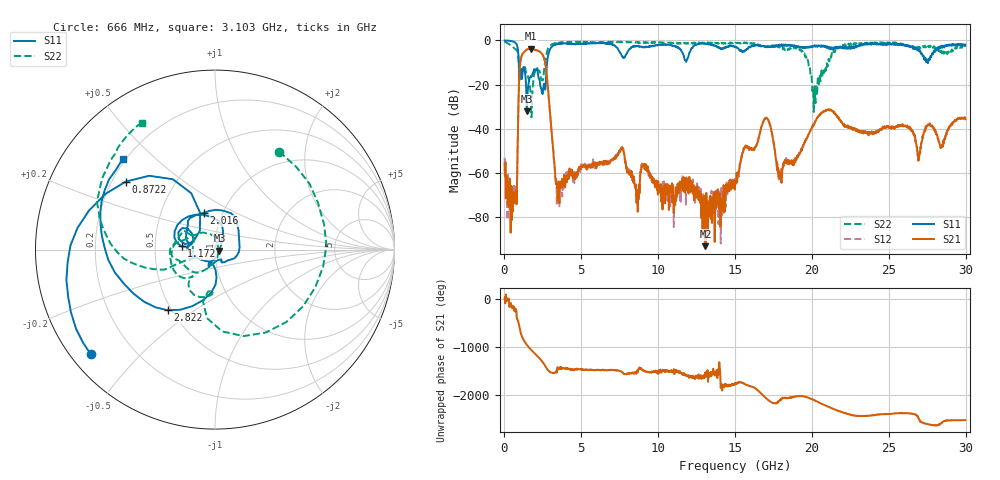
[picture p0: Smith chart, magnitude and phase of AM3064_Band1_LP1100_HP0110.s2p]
# Hz S DB R 50.0
!freq dBS11 angS11 dBS21 angS21 dBS12 angS12 dBS22 angS22
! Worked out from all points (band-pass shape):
!   1600 points, 10 MHz to 29.98 GHz, reference 50 ohm
!   highest |S21| = -3.79 dB at 1.697 GHz (marker M1); lowest = -93.0 dB at 13.07 GHz (marker M2)
!   |S21| within 3 dB of the highest: 1.133 GHz to 2.5 GHz (1.367 GHz wide, 75.3 % of centre)
!   lowest |S11| = -32.0 dB at 1.453 GHz (marker M3), VSWR 1.05, Z = 52.5 - j0.593 ohm
!   |S11| at or under -10 dB: 931.6 MHz to 2.776 GHz (1.844 GHz wide, 99.5 % of centre); 27.52257 GHz to 27.55001 GHz (27.45 MHz wide, 0.0997 % of centre)
!   |S22| runs from -34.8 to -0.5 dB; largest |S21 - S12| = 0.0097
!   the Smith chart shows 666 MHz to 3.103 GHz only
!   S11 on the Smith chart (normalised r, x): 666 MHz: 0.06, -0.36; 872.2 MHz: 0.26, +0.32; 1.172 GHz: 0.69, +0.03; 2.016 GHz: 0.82, +0.35; 2.822 GHz: 0.48, -0.39; 3.103 GHz: 0.19, +0.40
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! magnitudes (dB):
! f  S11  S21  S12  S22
! 10 MHz  0.0  -55.6  -53.0  -0.5
! 666 MHz  -0.9  -69.5  -70.1  -3.7
! 872.2 MHz  -4.1  -42.0  -42.1  -5.9
! 1.172 GHz  -14.6  -6.2  -6.1  -13.4
! 1.453 GHz  -32.0  -4.2  -4.1  -15.9
! 1.697 GHz  -16.2  -3.8  -3.8  -23.6
! 2.016 GHz  -13.4  -4.3  -4.2  -13.5
! 2.822 GHz  -7.4  -21.0  -20.9  -3.9
! 3.103 GHz  -2.8  -44.6  -44.2  -1.8
! 3.478 GHz  -1.7  -67.1  -66.8  -1.0
! 5.015 GHz  -1.5  -57.3  -56.5  -0.7
! 7.601 GHz  -6.6  -48.7  -48.8  -0.7
! 8.632 GHz  -2.6  -68.3  -68.1  -1.0
! 10 GHz  -2.1  -63.6  -65.5  -1.0
! 13.07 GHz  -1.4  -93.0  -72.6  -1.1
! 15 GHz  -2.9  -64.8  -64.7  -1.4
! 16.97 GHz  -2.8  -35.2  -35.2  -2.6
! 17.93 GHz  -2.1  -60.3  -60.1  -2.7
! 19.99 GHz  -3.1  -39.6  -39.5  -18.0
! 25 GHz  -1.3  -39.5  -39.3  -1.2
! 26.94 GHz  -4.4  -53.6  -51.8  -3.3
! 29.98 GHz  -1.9  -35.7  -35.4  -2.9
